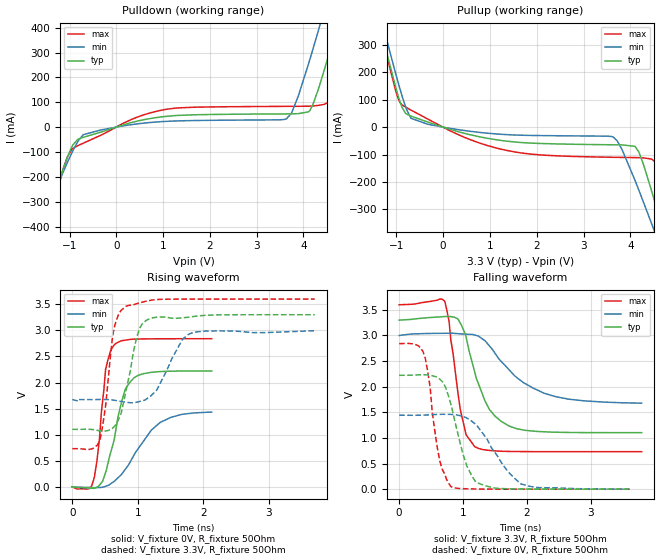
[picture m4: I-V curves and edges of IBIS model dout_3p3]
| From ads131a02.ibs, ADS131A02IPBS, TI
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|   dout_3p3 Model
[Model]   dout_3p3
Model_type   Output
Polarity   Non-Inverting
Vmeas = 1.65
Vref = 0
Cref = 2pF
Rref = 70
|   typ   min   max
|   (nom PVT)   (fast PVT)   (slow PVT)
C_comp   1.667e-12   1.601e-12   1.775e-12
| Where nom  PVT is Nominal Process, 3.3V, 27C
|   Fast PVT is Strong Process,  3.6V, -40C
|   Slow PVT is Weak Process,   3V, 125C
[Voltage Range]   3.3   3   3.6
|Junction Temperature
[Temperature Range]   27   125   -40
[Pullup Reference]   3.3   3   3.6
[Pulldown Reference]   0   0   0
[Power Clamp Reference]   3.3   3   3.6
[GND Clamp Reference]   0   0   0
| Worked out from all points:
|   slope of the pulldown table from 0 to 0.495 V, typ, clamps not added: 19.1 ohm
|   slope of the pullup table from 0 to 0.495 V, typ, clamps not added: 20.5 ohm
|   falling waveform, V_fixture 3.3V, R_fixture 50Ohm: 20-80 % time 356ps typ, 695ps min, 204ps max; typ from 3.3 V to 1.1 V
|   rising waveform, V_fixture 0V, R_fixture 50Ohm: 20-80 % time 244ps typ, 480ps min, 130ps max; typ from 0 V to 2.22 V
|   rising waveform, V_fixture 3.3V, R_fixture 50Ohm: 20-80 % time 213ps typ, 317ps min, 156ps max; typ from 1.1 V to 3.3 V
|   falling waveform, V_fixture 0V, R_fixture 50Ohm: 20-80 % time 280ps typ, 476ps min, 184ps max; typ from 2.22 V to 0 V
[Pulldown]
|   Voltage   I(typ)   I(min)   I(max)
-3.3V     -1.502A    -1.179A    -1.903A
-1.68V    -492mA     -424.5mA   -584.9mA
-1.324V   -276.6mA   -263.1mA   -304.4mA
-1.036V   -115.8mA   -138.2mA   -116.3mA
-705mV    -40.87mA   -30.17mA   -64.48mA
1.056V    43.13mA    23.1mA     71.26mA
3.633V    53.22mA    32.89mA    83.52mA
4.109V    61.66mA    255.1mA    84.15mA
4.329V    158.8mA    395.1mA    87.72mA
4.653V    365.5mA    608.1mA    162.3mA
5.161V    711.7mA    950.4mA    503.3mA
6.6V      1.731A     1.944A     1.55A
[Pullup]
|   Voltage   I(typ)   I(min)   I(max)
-3.3V     1.781A     1.774A     1.82A
-1.561V   518.9mA    556.1mA    518.6mA
-1.254V   304.1mA    349.6mA    294.7mA
-881.1mV  72.82mA    115.2mA    81.69mA
-690mV    40.36mA    32.34mA    62.35mA
-330mV    18.63mA    10.6mA     29.65mA
1.362V    -51.26mA   -27.38mA   -85.17mA
3.634V    -64.5mA    -36.24mA   -110.1mA
4.101V    -70.41mA   -195.1mA   -111.2mA
4.523V    -273mA     -383.6mA   -125.3mA
4.976V    -547.5mA   -592.2mA   -437.3mA
6.6V      -1.559A    -1.351A    -1.75A
[Ramp]
R_load = 50
|   typ   min   max
dV/dt_r   1.33397/2.37857e-10   0.866022/4.65421e-10   1.70408/1.40178e-10
dV/dt_f   1.31853/3.48217e-10   0.796423/6.5135e-10   1.72111/1.86588e-10
[Falling Waveform]
V_fixture = 3.3V
V_fixture_min = 3V
V_fixture_max = 3.6V
R_fixture = 50Ohm
|   Time   V(typ)   V(min)   V(max)
0s        3.3V       3V         3.6V
714.7ps   3.37V      3.043V     3.667V
781.2ps   3.371V     3.043V     3.283V
959.2ps   3.238V     3.031V     1.544V
1.048ns   2.971V     3.025V     1.062V
1.182ns   2.293V     3.01V      830.4mV
1.411ns   1.562V     2.801V     756.4mV
1.719ns   1.234V     2.334V     736.7mV
2.451ns   1.112V     1.806V     732mV
3.797ns   1.103V     1.679V     731.4mV
[Rising Waveform]
V_fixture = 0V
V_fixture_min = 0V
V_fixture_max = 0V
R_fixture = 50Ohm
|   Time   V(typ)   V(min)   V(max)
0s        750.8pV    33.66nV    199.1pV
256.4ps   -23.53mV   -11.57mV   -37.4mV
337.3ps   -29.58mV   -16.02mV   182.6mV
414.7ps   31.97mV    -13.22mV   909.5mV
508.2ps   273.1mV    9.834mV    2.247V
659.2ps   1.044V     126.5mV    2.744V
809.7ps   1.871V     335.4mV    2.811V
942.4ps   2.089V     607.7mV    2.831V
1.342ns   2.209V     1.234V     2.839V
2.13ns    2.222V     1.432V     2.84V
[Rising Waveform]
V_fixture = 3.3V
V_fixture_min = 3V
V_fixture_max = 3.6V
R_fixture = 50Ohm
|   Time   V(typ)   V(min)   V(max)
0s        1.102V     1.673V     731.4mV
419.5ps   1.072V     1.674V     882.6mV
512.4ps   1.071V     1.674V     1.586V
639.4ps   1.154V     1.66V      3.049V
818.6ps   1.831V     1.622V     3.459V
1.029ns   3.042V     1.636V     3.528V
1.178ns   3.223V     1.722V     3.572V
1.686ns   3.241V     2.834V     3.599V
1.847ns   3.265V     2.961V     3.6V
3.703ns   3.3V       2.993V     3.6V
[Falling Waveform]
V_fixture = 0V
V_fixture_min = 0V
V_fixture_max = 0V
R_fixture = 50Ohm
|   Time   V(typ)   V(min)   V(max)
0s        2.223V     1.443V     2.84V
374.2ps   2.234V     1.445V     2.685V
486.2ps   2.222V     1.452V     1.981V
518.6ps   2.213V     1.454V     1.499V
637.3ps   2.147V     1.461V     547mV
808.2ps   1.664V     1.46V      49.51mV
994.9ps   704.8mV    1.419V     9.975mV
1.198ns   142.2mV    1.268V     3.316mV
1.907ns   3.299mV    101.5mV    300.1uV
3.609ns   250.4uV    1.418mV    -148.9uV
